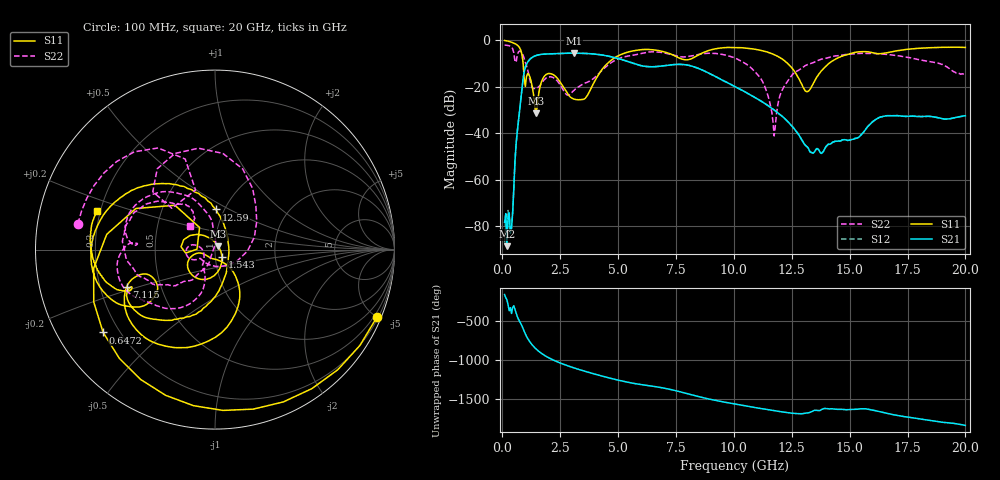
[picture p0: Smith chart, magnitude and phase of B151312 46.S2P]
!  2-Port S-parameters saved by WinCal
! VAR MeasName=S-Parameters (CALIBRATED_DATA) read from VNA (N5244A)
! VAR MeasDate=12/8/2015 5:47:27 PM
! VAR NAME=B151312 46
! VAR FILENAME=B151312 46.S2P
! VAR DATE=12/8/2015 5:47:27 PM
! VAR PHYS_PORTS=1,2
# Hz S DB R 50
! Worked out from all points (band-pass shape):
!   401 points, 100 MHz to 20 GHz, reference 50 ohm
!   highest |S21| = -5.65 dB at 3.085 GHz (marker M1); lowest = -88.5 dB at 199.5 MHz (marker M2)
!   |S21| within 3 dB of the highest: 1.161 GHz to 5.232 GHz (4.071 GHz wide, 127 % of centre)
!   lowest |S11| = -31.5 dB at 1.443 GHz (marker M3), VSWR 1.05, Z = 51.8 + j2 ohm
!   |S11| at or under -10 dB: 899.2 MHz to 4.549 GHz (3.65 GHz wide, 134 % of centre); 12.31 GHz to 14.12 GHz (1.801 GHz wide, 13.6 % of centre)
!   |S22| runs from -41.2 to -2.2 dB; largest |S21 - S12| = 0.0017
!   S11 on the Smith chart (normalised r, x): 100 MHz: 0.29, -4.99; 647.2 MHz: 0.14, -0.32; 1.543 GHz: 1.08, -0.09; 7.115 GHz: 0.32, -0.18; 12.59 GHz: 0.91, +0.43; 20 GHz: 0.19, +0.15
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1e8  -0.20 -22.6  -78.27 -159.0  -86.97 157.6  -2.19 169.3
1.995e8  -0.38 -44.4  -88.51 134.5  -84.16 95.3  -2.28 158.2
3.985e8  -0.94 -87.2  -80.78 -42.8  -80.54 18.1  -3.02 129.6
6.4725e8  -2.21 -143.5  -39.34 -82.3  -39.29 -82.4  -6.49 137.0
9.955e8  -19.95 178.8  -11.65 54.7  -11.65 54.6  -9.55 46.8
1.14475e9  -14.75 162.4  -8.83 -27.4  -8.83 -27.4  -14.85 -2.7
1.44325e9  -31.47 46.4  -6.72 -134.6  -6.72 -134.6  -20.72 -140.2
1.54275e9  -25.02 -45.7  -6.42 -161.2  -6.42 -161.2  -20.38 -149.4
2.13975e9  -14.61 -142.3  -5.92 87.2  -5.91 87.2  -15.92 -179.3
3.085e9  -25.33 -134.6  -5.65 -21.6  -5.65 -21.6  -21.77 -137.8
3.43325e9  -25.55 -101.1  -5.72 -54.0  -5.72 -54.0  -19.16 -129.2
4.72675e9  -8.51 -72.5  -7.27 -160.2  -7.25 -160.2  -9.57 -114.8
6.7665e9  -4.56 -148.3  -11.29 88.7  -11.29 88.6  -5.19 -172.0
7.11475e9  -5.45 -157.2  -10.92 69.4  -10.89 69.2  -5.82 179.8
1.005e10  -3.20 -178.2  -20.03 -128.1  -19.99 -128.4  -7.76 128.2
1.119425e10  -4.53 149.8  -26.33 173.5  -26.35 173.0  -17.03 95.5
1.17415e10  -6.31 130.6  -30.02 147.2  -30.09 147.0  -41.17 147.2
1.258725e10  -13.00 88.5  -37.84 112.6  -37.84 112.7  -14.32 -125.9
1.338325e10  -19.56 -47.8  -48.36 137.9  -48.48 138.5  -9.89 -141.5
1.45275e10  -7.52 -114.8  -43.34 163.7  -43.41 164.1  -6.71 -165.1
1.67165e10  -5.28 -154.9  -32.54 104.8  -32.44 104.4  -6.29 153.1
2e10  -3.21 162.0  -32.58 -43.0  -32.67 -43.4  -14.45 136.3
